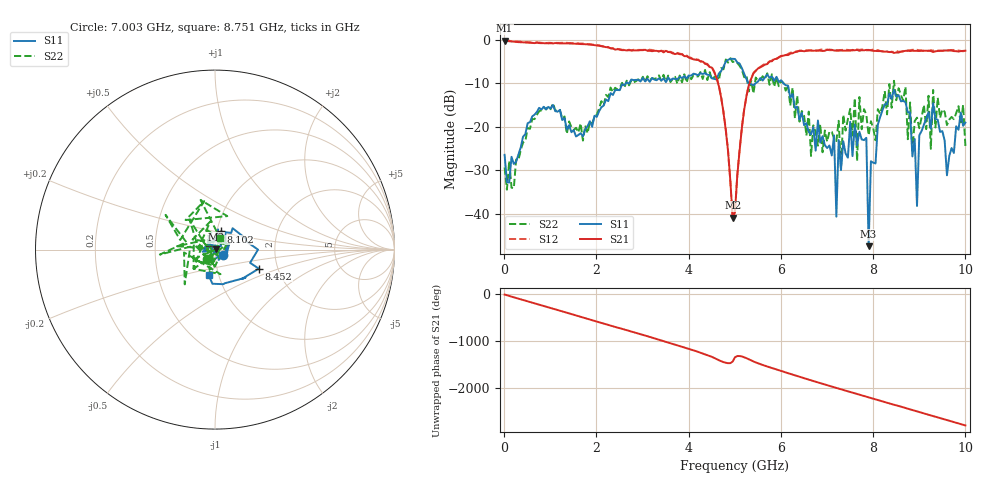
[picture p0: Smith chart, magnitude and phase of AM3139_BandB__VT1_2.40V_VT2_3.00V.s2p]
! Date/Time: Tue, Nov 13, 2018 5:00 PM
! Network Analyzer: Agilent Technologies E8364B Rev: A.07.50.67
! Sweep from 0.010 to 10.000 GHz, 201 Points, Sweep Type: LIN
! Power Supply: 2.401 V, 0.000 A
# Hz S DB R 50
!freq MagS11 AngS11 MagS21 AngS21 MagS12 AngS12 MagS22 AngS22
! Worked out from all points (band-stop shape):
!   201 points, 10 MHz to 10 GHz, reference 50 ohm
!   highest |S21| = -0.26 dB at 10 MHz (marker M1); lowest = -40.9 dB at 4.955 GHz (marker M2)
!   |S21| within 3 dB of the highest: start of sweep to 3.683 GHz; 6.2 GHz to end of sweep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
!   lowest |S11| = -47.4 dB at 7.902 GHz (marker M3), VSWR 1.01, Z = 50.4 + j0.206 ohm
!   |S11| at or under -10 dB: start of sweep to 2.644 GHz; 5.297 GHz to 5.456 GHz (159.3 MHz wide, 2.96 % of centre); 6.052 GHz to end of sweep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
!   |S22| runs from -34.4 to -4.3 dB; largest |S21 - S12| = 0.033
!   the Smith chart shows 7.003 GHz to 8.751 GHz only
!   S11 on the Smith chart (normalised r, x): 7.003 GHz: 1.09, -0.07; 8.102 GHz: 1.04, +0.21; 8.452 GHz: 1.60, -0.36; 8.751 GHz: 0.90, -0.26
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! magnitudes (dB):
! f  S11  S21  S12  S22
! 10 MHz  -26.5  -0.3  -0.3  -29.3
! 1.708 GHz  -22.2  -1.0  -1.0  -23.2
! 3.357 GHz  -8.9  -2.7  -2.7  -8.2
! 4.555 GHz  -9.0  -7.5  -7.4  -8.6
! 4.955 GHz  -4.4  -40.9  -41.3  -5.2
! 5.005 GHz  -4.5  -39.5  -39.4  -5.0
! 5.405 GHz  -10.5  -7.7  -7.7  -12.4
! 6.703 GHz  -20.1  -2.6  -2.5  -19.7
! 7.003 GHz  -24.9  -2.4  -2.3  -23.4
! 7.153 GHz  -22.0  -2.5  -2.5  -22.8
! 7.203 GHz  -40.6  -2.5  -2.4  -23.3
! 7.253 GHz  -23.0  -2.6  -2.4  -18.6
! 7.852 GHz  -22.5  -2.4  -2.5  -17.3
! 7.902 GHz  -47.4  -2.4  -2.5  -22.0
! 8.102 GHz  -19.5  -2.6  -2.4  -16.0
! 8.352 GHz  -12.4  -2.9  -2.9  -10.2
! 8.452 GHz  -11.5  -3.1  -2.8  -9.5
! 8.751 GHz  -16.7  -2.6  -2.5  -22.9
! 8.951 GHz  -38.2  -2.6  -2.3  -17.9
! 9.301 GHz  -14.6  -2.8  -2.5  -11.6
! 9.6 GHz  -31.1  -2.5  -2.5  -19.6
! 10 GHz  -19.1  -2.6  -2.5  -24.5
